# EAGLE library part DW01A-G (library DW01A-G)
One Cell Lithium-ion/Polymer Battery Protection IC Source: Datasheet
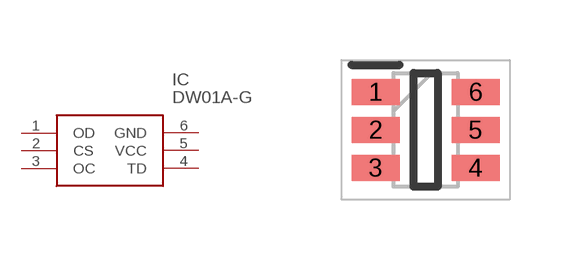
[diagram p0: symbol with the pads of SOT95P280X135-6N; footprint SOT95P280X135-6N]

Designator prefix IC

## DW01A-G (Description: One Cell Lithium-ion/Polymer Battery Protection IC; Height: 1.35mm; Manufacturer_Name: Fortune Semiconductor Corporation; Manufacturer_Part_Number: DW01A-G)  [SOT95P280X135-6N]
1  OD
2  CS
3  OC
4  TD
5  VCC
6  GND

## Footprint SOT95P280X135-6N (pad centres in mm)
DW01A-G
smd 1.2 x 0.65: 1 -1.25,0.95; 2 -1.25,0; 3 -1.25,-0.95; 4 1.25,-0.95; 5 1.25,0; 6 1.25,0.95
